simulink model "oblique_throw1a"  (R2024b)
settings: Solver=VariableStepAuto  StartTime=0.0  StopTime=3  RelTol=1e-3

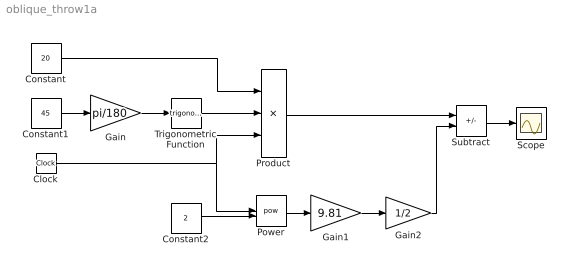
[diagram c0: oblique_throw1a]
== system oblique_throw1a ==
  Clock : Clock
  Constant : Constant  Value=20
  Constant1 : Constant  Value=45
  Constant2 : Constant  Value=2
  Gain : Gain  Gain=pi/180
  Gain1 : Gain  Gain=9.81
  Gain2 : Gain  Gain=1/2
  Power : Math  Operator=pow
  Product : Product  Inputs=3
  Scope : Scope
  Subtract : Sum  Inputs=+-
  Trigonometric Function : Trigonometry
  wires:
  Constant1/1 -> Gain/1
  Gain/1 -> Trigonometric Function/1
  Trigonometric Function/1 -> Product/2
  Clock/1 -> Power/1, Product/3
  Constant/1 -> Product/1
  Constant2/1 -> Power/2
  Power/1 -> Gain1/1
  Gain1/1 -> Gain2/1
  Product/1 -> Subtract/1
  Gain2/1 -> Subtract/2
  Subtract/1 -> Scope/1
